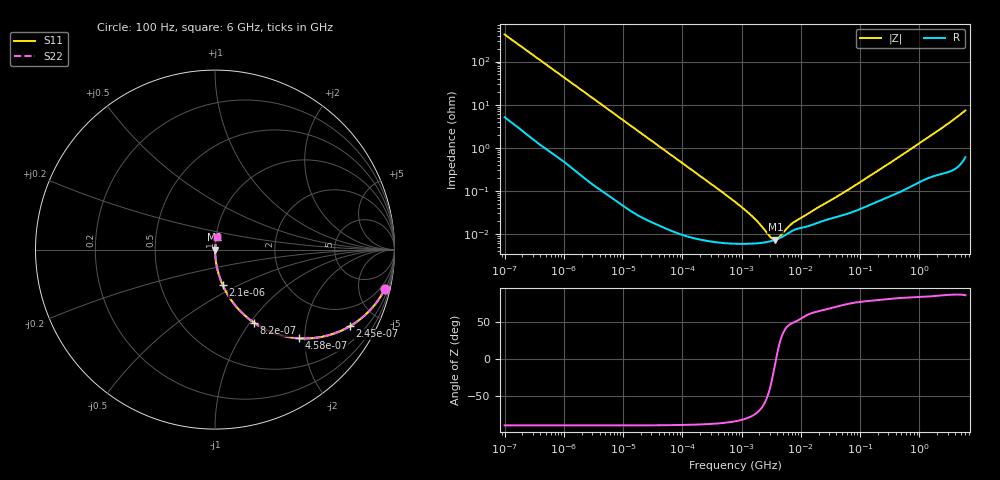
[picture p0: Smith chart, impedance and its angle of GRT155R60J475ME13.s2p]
!Murata Part Number: GRT155R60J475ME13
!These Parameters are Measured in Series Mode Connection
!Data Generated on Jun 19, 2026
!  o--ll--o
!Port1  Port2
!  o------o
!Operation Temp=25[degC], DC Bias Voltage=0[V]
!Freq. Start=100[Hz] Stop=6[GHz] 401[Steps]
# Hz S RI R 50
!Freq.(Hz) S11(Real) S11(Imag) S21(Real) S21(Imag) S12(Real) S12(Imag) S22(Real) S22(Imag)
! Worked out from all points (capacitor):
!   401 points, 100 Hz to 6 GHz, reference 50 ohm
!   read as one part in series: C = 3.74 uF near 109 Hz
!   lowest |Z| = 7.32 mohm at 3.712 MHz (marker M1)
!   series resonance near 3.829 MHz, so ESL is about 460 pH
!   S11 on the Smith chart (normalised r, x): 100 Hz: 1.10, -8.48; 245 Hz: 1.04, -3.49; 458 Hz: 1.02, -1.87; 820 Hz: 1.01, -1.05; 2.1 kHz: 1.00, -0.41; 6 GHz: 1.01, +0.15
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100  0.9449 -0.2223  0.0551 0.2223  0.0551 0.2223  0.9449 -0.2223
164  0.8683 -0.3324  0.1317 0.3324  0.1317 0.3324  0.8683 -0.3324
245  0.75 -0.4274  0.25 0.4274  0.25 0.4274  0.75 -0.4274
350  0.5976 -0.485  0.4024 0.485  0.4024 0.485  0.5976 -0.485
458  0.4669 -0.4935  0.5331 0.4935  0.5331 0.4935  0.4669 -0.4935
820  0.2184 -0.4077  0.7816 0.4077  0.7816 0.4077  0.2184 -0.4077
1227  0.1127 -0.3109  0.8873 0.3109  0.8873 0.3109  0.1127 -0.3109
2008  0.0463 -0.2052  0.9537 0.2052  0.9537 0.2052  0.0463 -0.2052
2100  0.0426 -0.197  0.9574 0.197  0.9574 0.197  0.0426 -0.197
6728  0.00483 -0.0645  0.9952 0.0645  0.9952 0.0645  0.00483 -0.0645
40335  0.000276 -0.0109  0.9997 0.0109  0.9997 0.0109  0.000276 -0.0109
774597  5.93e-05 -0.000553  0.9999 0.000553  0.9999 0.000553  5.93e-05 -0.000553
1516199  5.94e-05 -0.000248  0.9999 0.000248  0.9999 0.000248  5.94e-05 -0.000248
2713602  6.5e-05 -8.1e-05  0.9999 8.1e-05  0.9999 8.1e-05  6.5e-05 -8.1e-05
3712478  7.29e-05 -7e-06  0.9999 7e-06  0.9999 7e-06  7.29e-05 -7e-06
4856642  8.56e-05 5.3e-05  0.9999 -5.3e-05  0.9999 -5.3e-05  8.56e-05 5.3e-05
7266822  0.000119 0.000133  0.9999 -0.000133  0.9999 -0.000133  0.000119 0.000133
1.555665e7  0.000162 0.000298  0.9998 -0.000298  0.9998 -0.000298  0.000162 0.000298
5.449875e7  0.00028 0.00089  0.9997 -0.00089  0.9997 -0.00089  0.00028 0.00089
3.124326e8  0.000748 0.00428  0.9993 -0.00428  0.9993 -0.00428  0.000748 0.00428
1.95892e9  0.00283 0.0233  0.9972 -0.0233  0.9972 -0.0233  0.00283 0.0233
6e9  0.0112 0.0716  0.9888 -0.0716  0.9888 -0.0716  0.0112 0.0716
